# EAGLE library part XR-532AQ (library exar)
PULSE DETECTOR
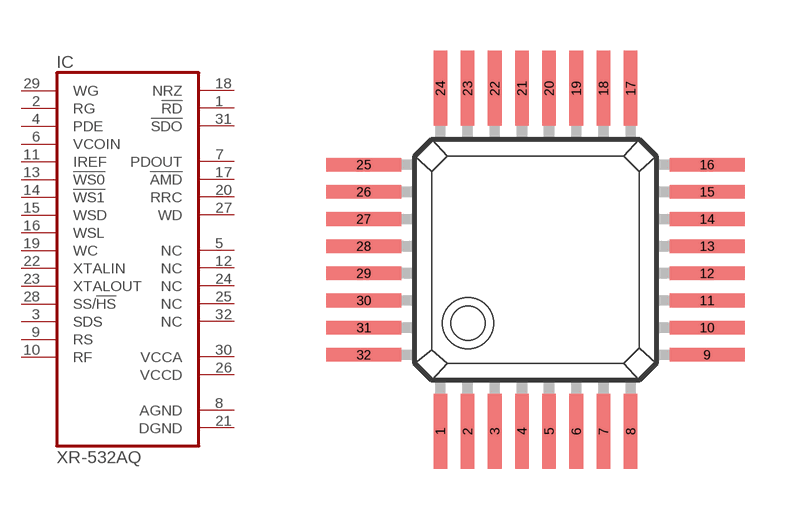
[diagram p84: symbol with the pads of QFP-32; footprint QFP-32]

Designator prefix IC

## XR-532AQ (OC_FARNELL: unknown; OC_NEWARK: unknown)  [QFP-32]
1  !RD
2  RG  in
3  SDS  in
4  PDE  in
5  NC  nc
6  VCOIN  in
7  PDOUT  out
8  AGND  pwr
9  RS  in
10  RF  in
11  IREF  in
12  NC  nc
13  !WS0  in
14  !WS1  in
15  WSD  in
16  WSL  in
17  !AMD  out
18  NRZ
19  WC  in
20  RRC  out
21  DGND  pwr
22  XTALIN  in
23  XTALOUT  in
24  NC  nc
25  NC  nc
26  VCCD  pwr
27  WD  out
28  SS/!HS  in
29  WG  in
30  VCCA  pwr
31  !SDO
32  NC  nc

## Footprint QFP-32 (pad centres in mm)
Quad Flat Package
smd 0.4 x 2.2: 1 -2.8,-5.05; 2 -2,-5.05; 3 -1.2,-5.05; 4 -0.4,-5.05; 5 0.4,-5.05; 6 1.2,-5.05; 7 2,-5.05; 8 2.8,-5.05; 17 2.8,5.05; 18 2,5.05; 19 1.2,5.05; 20 0.4,5.05; 21 -0.4,5.05; 22 -1.2,5.05; 23 -2,5.05; 24 -2.8,5.05
smd 2.2 x 0.4: 9 5.05,-2.8; 10 5.05,-2; 11 5.05,-1.2; 12 5.05,-0.4; 13 5.05,0.4; 14 5.05,1.2; 15 5.05,2; 16 5.05,2.8; 25 -5.05,2.8; 26 -5.05,2; 27 -5.05,1.2; 28 -5.05,0.4; 29 -5.05,-0.4; 30 -5.05,-1.2; 31 -5.05,-2; 32 -5.05,-2.8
